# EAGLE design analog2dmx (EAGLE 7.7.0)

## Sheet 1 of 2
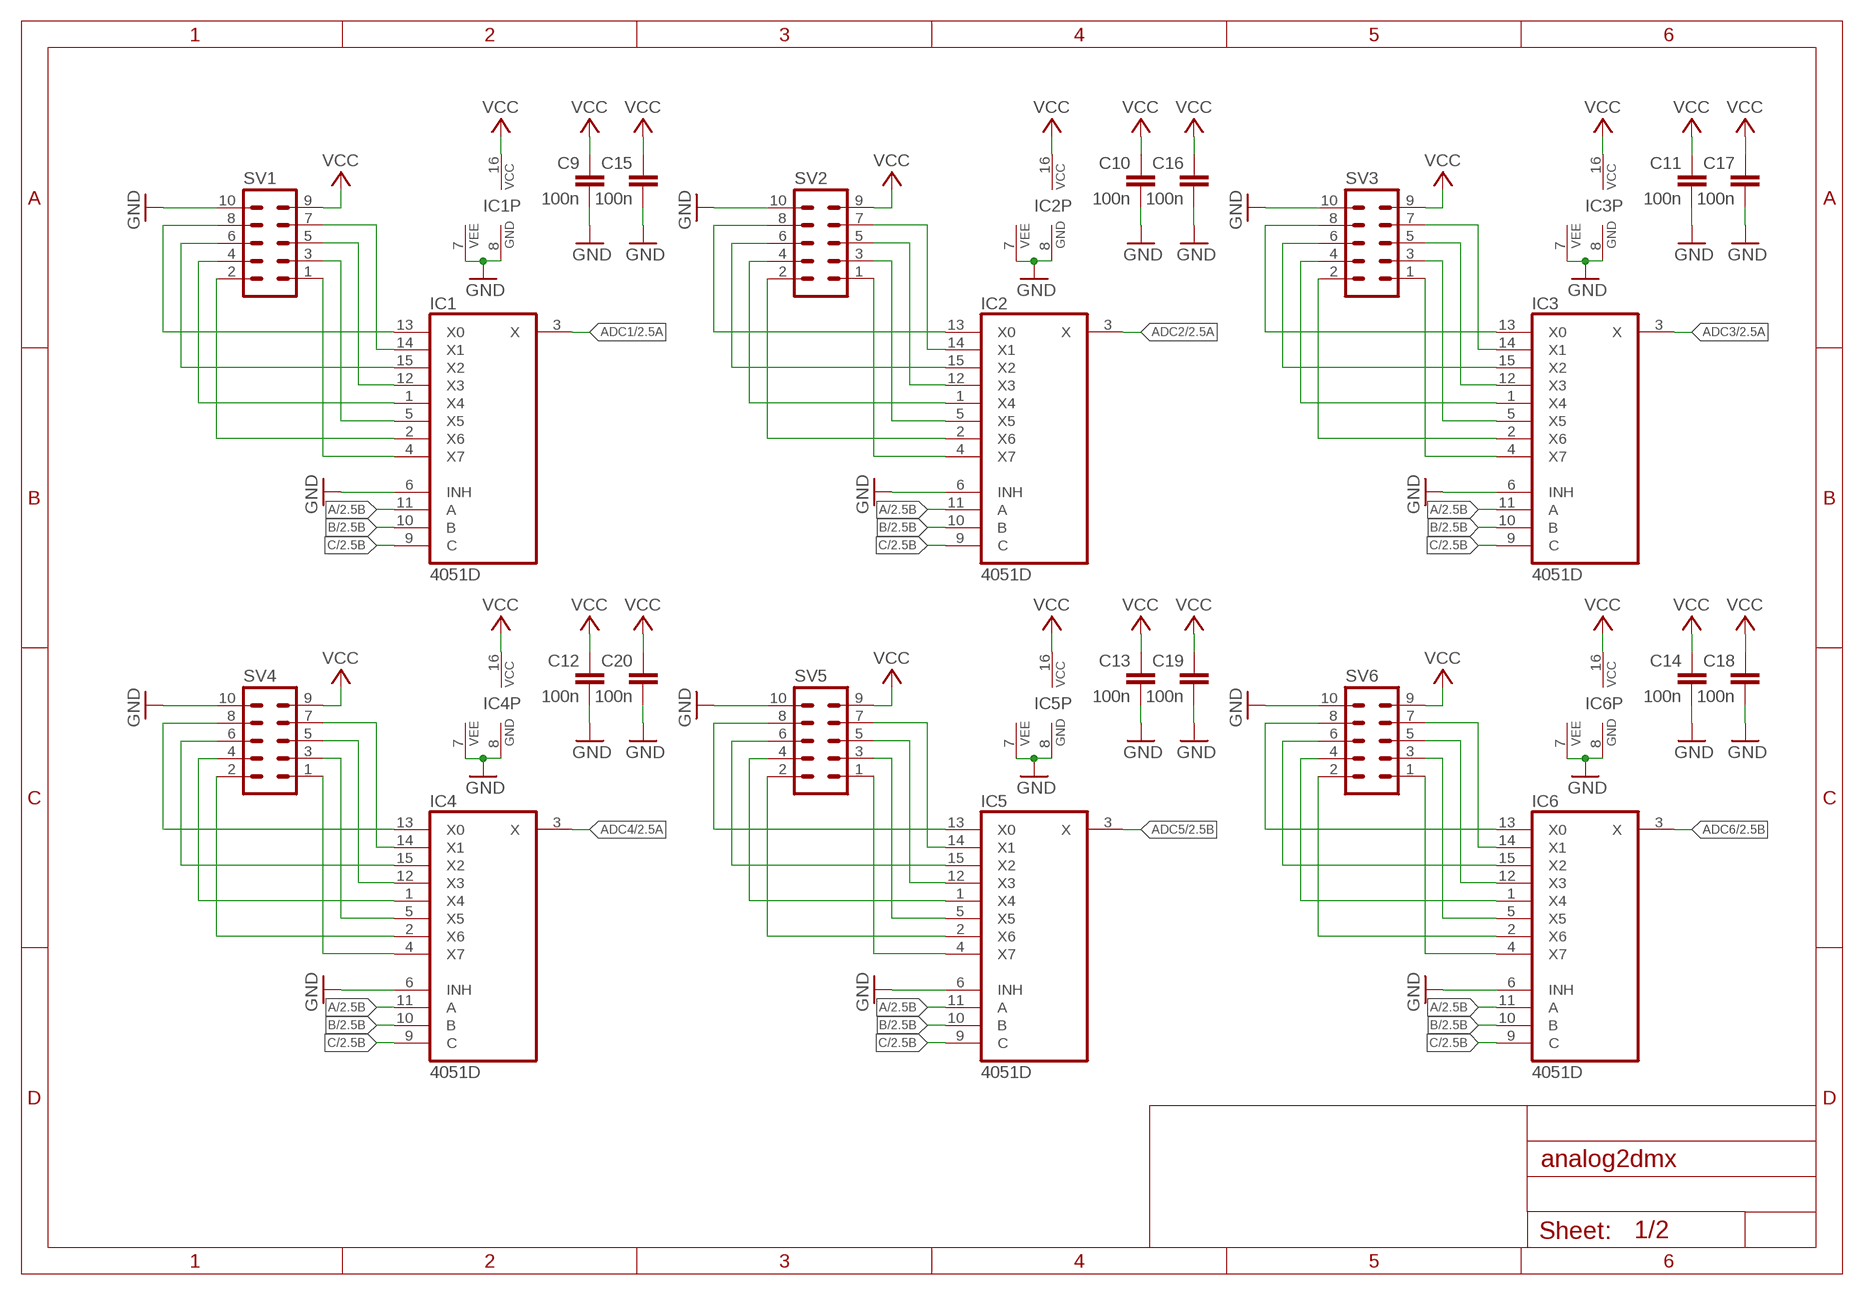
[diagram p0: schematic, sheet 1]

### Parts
C9  100n  C-EUC0603  [C0603]
C10  100n  C-EUC0603  [C0603]
C11  100n  C-EUC0603  [C0603]
C12  100n  C-EUC0603  [C0603]
C13  100n  C-EUC0603  [C0603]
C14  100n  C-EUC0603  [C0603]
C15  100n  C-EUC0603  [C0603]
C16  100n  C-EUC0603  [C0603]
C17  100n  C-EUC0603  [C0603]
C18  100n  C-EUC0603  [C0603]
C19  100n  C-EUC0603  [C0603]
C20  100n  C-EUC0603  [C0603]
IC1  4051D  [SO16]
IC2  4051D  [SO16]
IC3  4051D  [SO16]
IC4  4051D  [SO16]
IC5  4051D  [SO16]
IC6  4051D  [SO16]
SV1  ML10  [ML10]
SV2  ML10  [ML10]
SV3  ML10  [ML10]
SV4  ML10  [ML10]
SV5  ML10  [ML10]
SV6  ML10  [ML10]

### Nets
A: IC1.11(A) IC2.11(A) IC3.11(A) IC4.11(A) IC5.11(A) IC6.11(A) ; also sheet 2
ADC1: IC1.3(X) ; also sheet 2
ADC2: IC2.3(X) ; also sheet 2
ADC3: IC3.3(X) ; also sheet 2
ADC4: IC4.3(X) ; also sheet 2
ADC5: IC5.3(X) ; also sheet 2
ADC6: IC6.3(X) ; also sheet 2
B: IC1.10(B) IC2.10(B) IC3.10(B) IC4.10(B) IC5.10(B) IC6.10(B) ; also sheet 2
C: IC1.9(C) IC2.9(C) IC3.9(C) IC4.9(C) IC5.9(C) IC6.9(C) ; also sheet 2
GND: C9.2 C10.2 C11.2 C12.2 C13.2 C14.2 C15.2 C16.2 C17.2 C18.2 C19.2 C20.2 IC1.6(INH) IC1.7(VEE) IC1.8(GND) IC2.6(INH) IC2.7(VEE) IC2.8(GND) IC3.6(INH) IC3.7(VEE) IC3.8(GND) IC4.6(INH) IC4.7(VEE) IC4.8(GND) IC5.6(INH) IC5.7(VEE) IC5.8(GND) IC6.6(INH) IC6.7(VEE) IC6.8(GND) SV1.10 SV2.10 SV3.10 SV4.10 SV5.10 SV6.10 ; also sheet 2
N$1: IC1.4(X7) SV1.1
N$2: IC1.5(X5) SV1.3
N$3: IC1.12(X3) SV1.5
N$4: IC1.14(X1) SV1.7
N$5: IC1.2(X6) SV1.2
N$6: IC1.1(X4) SV1.4
N$7: IC1.15(X2) SV1.6
N$8: IC1.13(X0) SV1.8
N$9: IC2.4(X7) SV2.1
N$10: IC2.5(X5) SV2.3
N$11: IC2.12(X3) SV2.5
N$12: IC2.14(X1) SV2.7
N$13: IC2.2(X6) SV2.2
N$14: IC2.1(X4) SV2.4
N$15: IC2.15(X2) SV2.6
N$16: IC2.13(X0) SV2.8
N$17: IC3.4(X7) SV3.1
N$18: IC3.5(X5) SV3.3
N$19: IC3.12(X3) SV3.5
N$20: IC3.14(X1) SV3.7
N$21: IC3.2(X6) SV3.2
N$22: IC3.1(X4) SV3.4
N$23: IC3.15(X2) SV3.6
N$24: IC3.13(X0) SV3.8
N$25: IC4.4(X7) SV4.1
N$26: IC4.5(X5) SV4.3
N$27: IC4.12(X3) SV4.5
N$28: IC4.14(X1) SV4.7
N$29: IC4.2(X6) SV4.2
N$30: IC4.1(X4) SV4.4
N$31: IC4.15(X2) SV4.6
N$32: IC4.13(X0) SV4.8
N$33: IC5.4(X7) SV5.1
N$34: IC5.5(X5) SV5.3
N$35: IC5.12(X3) SV5.5
N$36: IC5.14(X1) SV5.7
N$37: IC5.2(X6) SV5.2
N$38: IC5.1(X4) SV5.4
N$39: IC5.15(X2) SV5.6
N$40: IC5.13(X0) SV5.8
N$41: IC6.4(X7) SV6.1
N$42: IC6.5(X5) SV6.3
N$43: IC6.12(X3) SV6.5
N$44: IC6.14(X1) SV6.7
N$45: IC6.2(X6) SV6.2
N$46: IC6.1(X4) SV6.4
N$47: IC6.15(X2) SV6.6
N$48: IC6.13(X0) SV6.8
VCC: C9.1 C10.1 C11.1 C12.1 C13.1 C14.1 C15.1 C16.1 C17.1 C18.1 C19.1 C20.1 IC1.16(VCC) IC2.16(VCC) IC3.16(VCC) IC4.16(VCC) IC5.16(VCC) IC6.16(VCC) SV1.9 SV2.9 SV3.9 SV4.9 SV5.9 SV6.9 ; also sheet 2

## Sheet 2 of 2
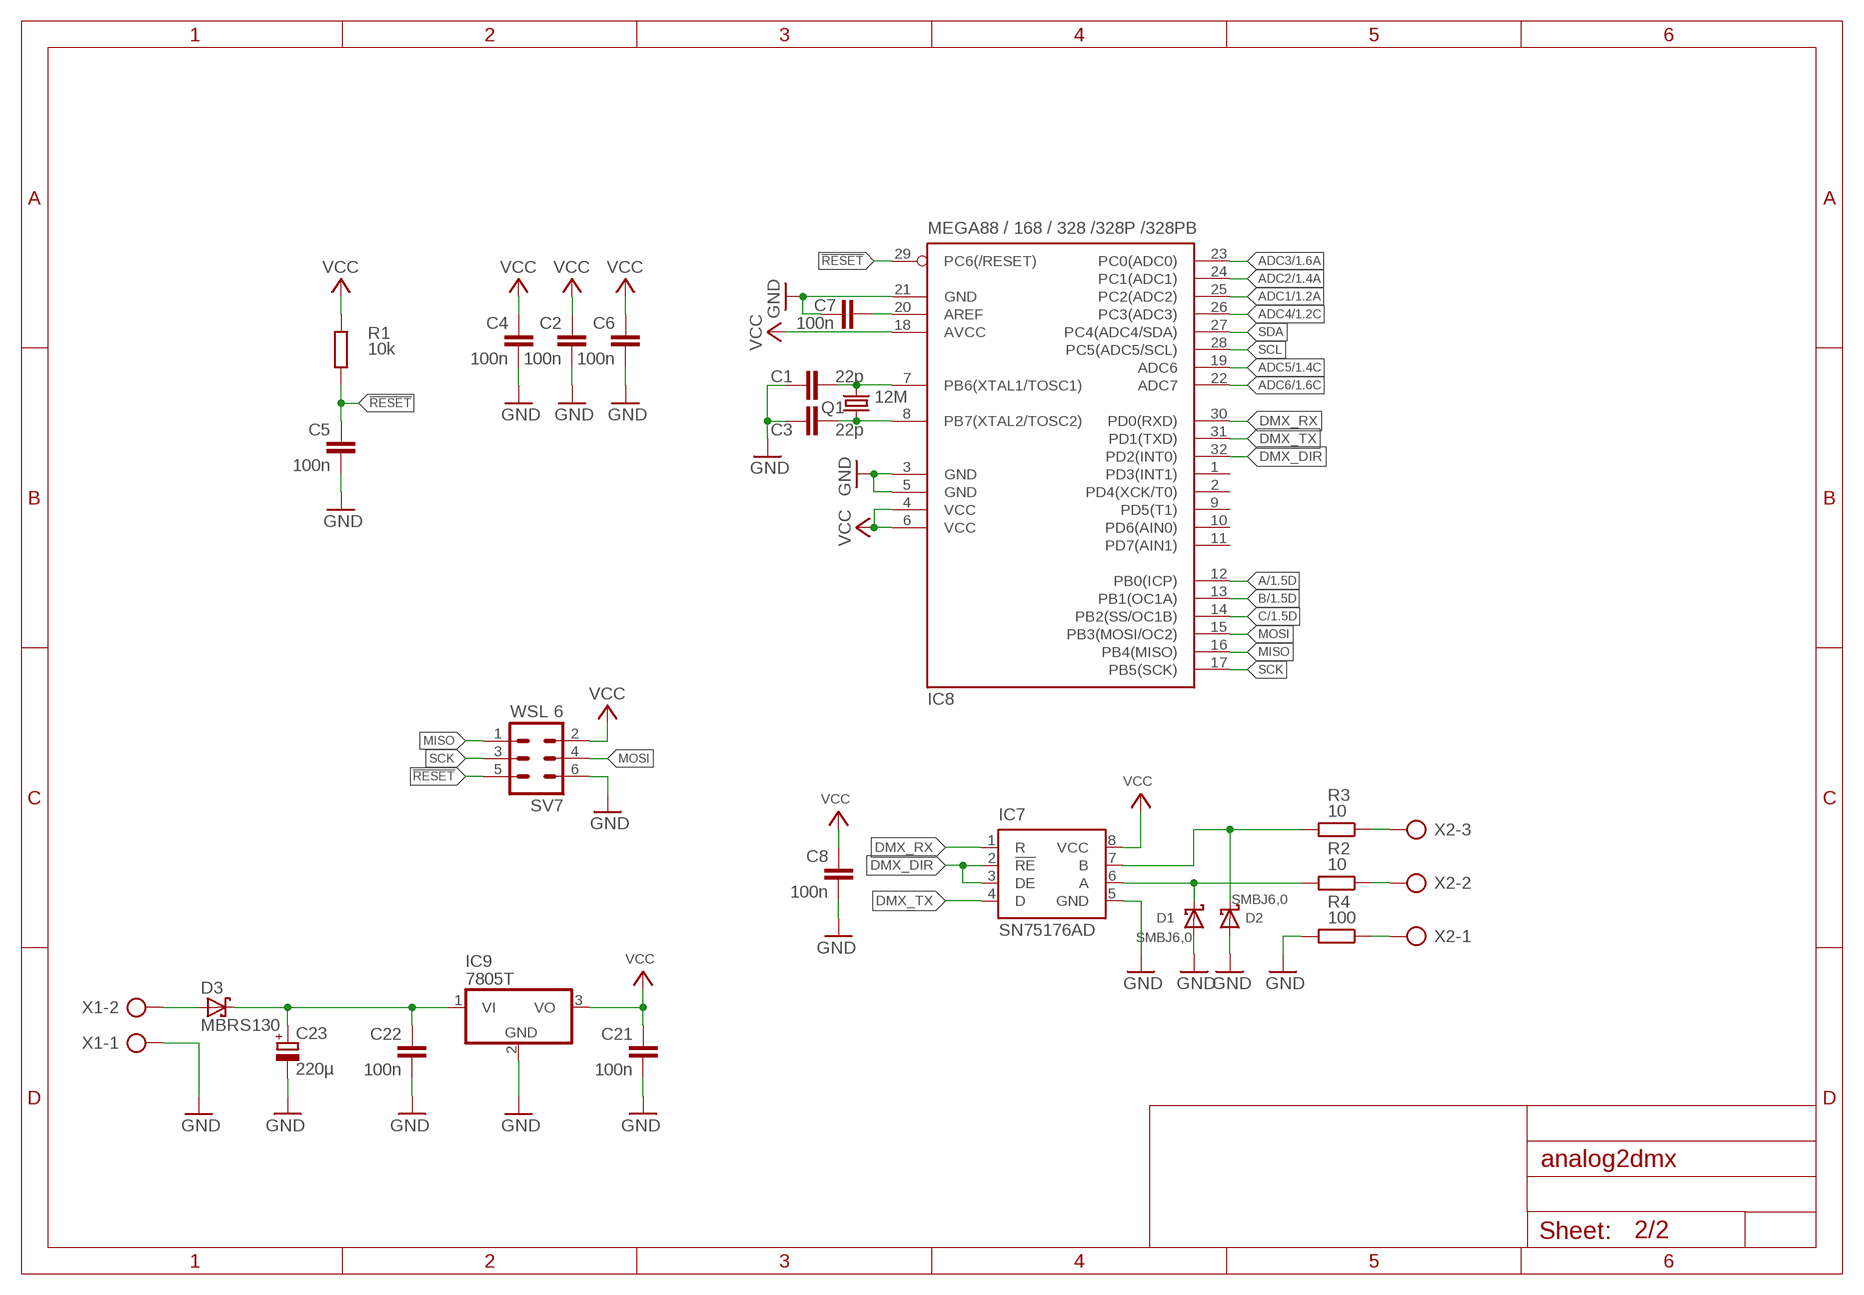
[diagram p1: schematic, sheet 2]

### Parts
C1  22p  C-EUC0603  [C0603]
C2  100n  C-EUC0603  [C0603]
C3  22p  C-EUC0603  [C0603]
C4  100n  C-EUC0603  [C0603]
C5  100n  C-EUC0603  [C0603]
C6  100n  C-EUC0603  [C0603]
C7  100n  C-EUC0603  [C0603]
C8  100n  C-EUC0603  [C0603]
C21  100n  C-EUC0603  [C0603]
C22  100n  C-EUC0603  [C0603]
C23  220µ  CPOL-EUE3.5-8  [E3,5-8]
D1  SMBJ6,0  MBRS130LT3  [SMB]
D2  SMBJ6,0  MBRS130LT3  [SMB]
D3  MBRS130  MBRS130LT3  [SMB]
IC7  SN75176AD  SN65176D  [SO-08]
IC8  MEGA88 / 168 / 328 /328P /328PB  MEGA8-AI  [TQFP32-08]
IC9  7805T  [TO220H]
Q1  12M  CRYSTALHC49S  [HC49/S]
R1  10k  R-EU_R0603  [R0603]
R2  10  R-EU_R0603  [R0603]
R3  10  R-EU_R0603  [R0603]
R4  100  R-EU_R0603  [R0603]
SV7  WSL 6  ML6  [ML6]
X1  AK500/2  [AK500/2]
X2  AK500/3  [AK500/3]

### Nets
!RESET: C5.1 IC8.29(PC6(/RESET)) R1.1 SV7.5
A: IC8.12(PB0(ICP)) ; also sheet 1
ADC1: IC8.25(PC2(ADC2)) ; also sheet 1
ADC2: IC8.24(PC1(ADC1)) ; also sheet 1
ADC3: IC8.23(PC0(ADC0)) ; also sheet 1
ADC4: IC8.26(PC3(ADC3)) ; also sheet 1
ADC5: IC8.19(ADC6) ; also sheet 1
ADC6: IC8.22(ADC7) ; also sheet 1
B: IC8.13(PB1(OC1A)) ; also sheet 1
C: IC8.14(PB2(SS/OC1B)) ; also sheet 1
DMX_DIR: IC7.2(!RE) IC7.3(DE) IC8.32(PD2(INT0))
DMX_RX: IC7.1(R) IC8.30(PD0(RXD))
DMX_TX: IC7.4(D) IC8.31(PD1(TXD))
GND: C1.1 C2.2 C3.1 C4.2 C5.2 C6.2 C7.1 C8.2 C21.2 C22.2 C23.- D1.A D2.A IC7.5(GND) IC8.3(GND) IC8.5(GND) IC8.21(GND) IC9.2(GND) R4.2 SV7.6 X1.1 ; also sheet 1
MISO: IC8.16(PB4(MISO)) SV7.1
MOSI: IC8.15(PB3(MOSI/OC2)) SV7.4
N$49: D2.C IC7.7(B) R3.2
N$50: D1.C IC7.6(A) R2.2
N$55: R3.1 X2.3
N$56: R2.1 X2.2
N$57: R4.1 X2.1
N$58: D3.A X1.2
N$59: C22.1 C23.+ D3.C IC9.1(VI)
N$65: C1.2 IC8.7(PB6(XTAL1/TOSC1)) Q1.2
N$66: C3.2 IC8.8(PB7(XTAL2/TOSC2)) Q1.1
N$67: C7.2 IC8.20(AREF)
SCK: IC8.17(PB5(SCK)) SV7.3
SCL: IC8.28(PC5(ADC5/SCL))
SDA: IC8.27(PC4(ADC4/SDA))
VCC: C2.1 C4.1 C6.1 C8.1 C21.1 IC7.8(VCC) IC8.4(VCC) IC8.6(VCC) IC8.18(AVCC) IC9.3(VO) R1.2 SV7.2 ; also sheet 1
Unconnected: IC8.1(PD3(INT1)) IC8.2(PD4(XCK/T0)) IC8.9(PD5(T1)) IC8.10(PD6(AIN0)) IC8.11(PD7(AIN1))

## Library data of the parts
C1-C22 = rcl:C-EU: CAPACITOR, European symbol
C23 = rcl:CPOL-EU: POLARIZED CAPACITOR, European symbol
D1-D3 = diode:MBRS130LT3: Schottky Power Rectifier
IC1-IC6 = 40xx:4051: 8-channel ANALOG MULTIPLEXER
IC7 = texas:SN65176: DIFFERENTIAL BUS TRANSCEIVER Source: http://focus.ti.com .. sn65176b.pdf
IC8 = atmel:MEGA8: MICROCONTROLLER 8 Kbytes FLASH, 1 kbytes SRAM, 512 bytes EEPROM, USART, 6-channel 10 bit ADC, 2-channel 8 bit ADC Pin compatible with Atmega48, ATMega88, ATMega168 Source: avr.lbr; MPN: ATMEGA8-16AU; OC_FARNELL: 9171371; OC_NEWARK: 73M8863
IC9 = linear:78*: Positive VOLTAGE REGULATOR Source: http://cache.national.com/ds/LM/LM78L05.pdf http://www.fairchildsemi.com/ds/LM/LM7805.pdf
Q1 = crystal:CRYSTAL: CRYSTAL; OC_FARNELL: 1667008; OC_NEWARK: unknown
R1-R4 = rcl:R-EU_: RESISTOR, European symbol
SV1-SV6 = con-harting-ml:ML10: HARTING; OC_FARNELL: unknown; OC_NEWARK: unknown
SV7 = con-harting-ml:ML6: HARTING; OC_FARNELL: unknown; OC_NEWARK: unknown
X1 = con-ptr500:AK500/2: CONNECTOR; OC_FARNELL: unknown; OC_NEWARK: unknown
X2 = con-ptr500:AK500/3: CONNECTOR; OC_FARNELL: unknown; OC_NEWARK: unknown

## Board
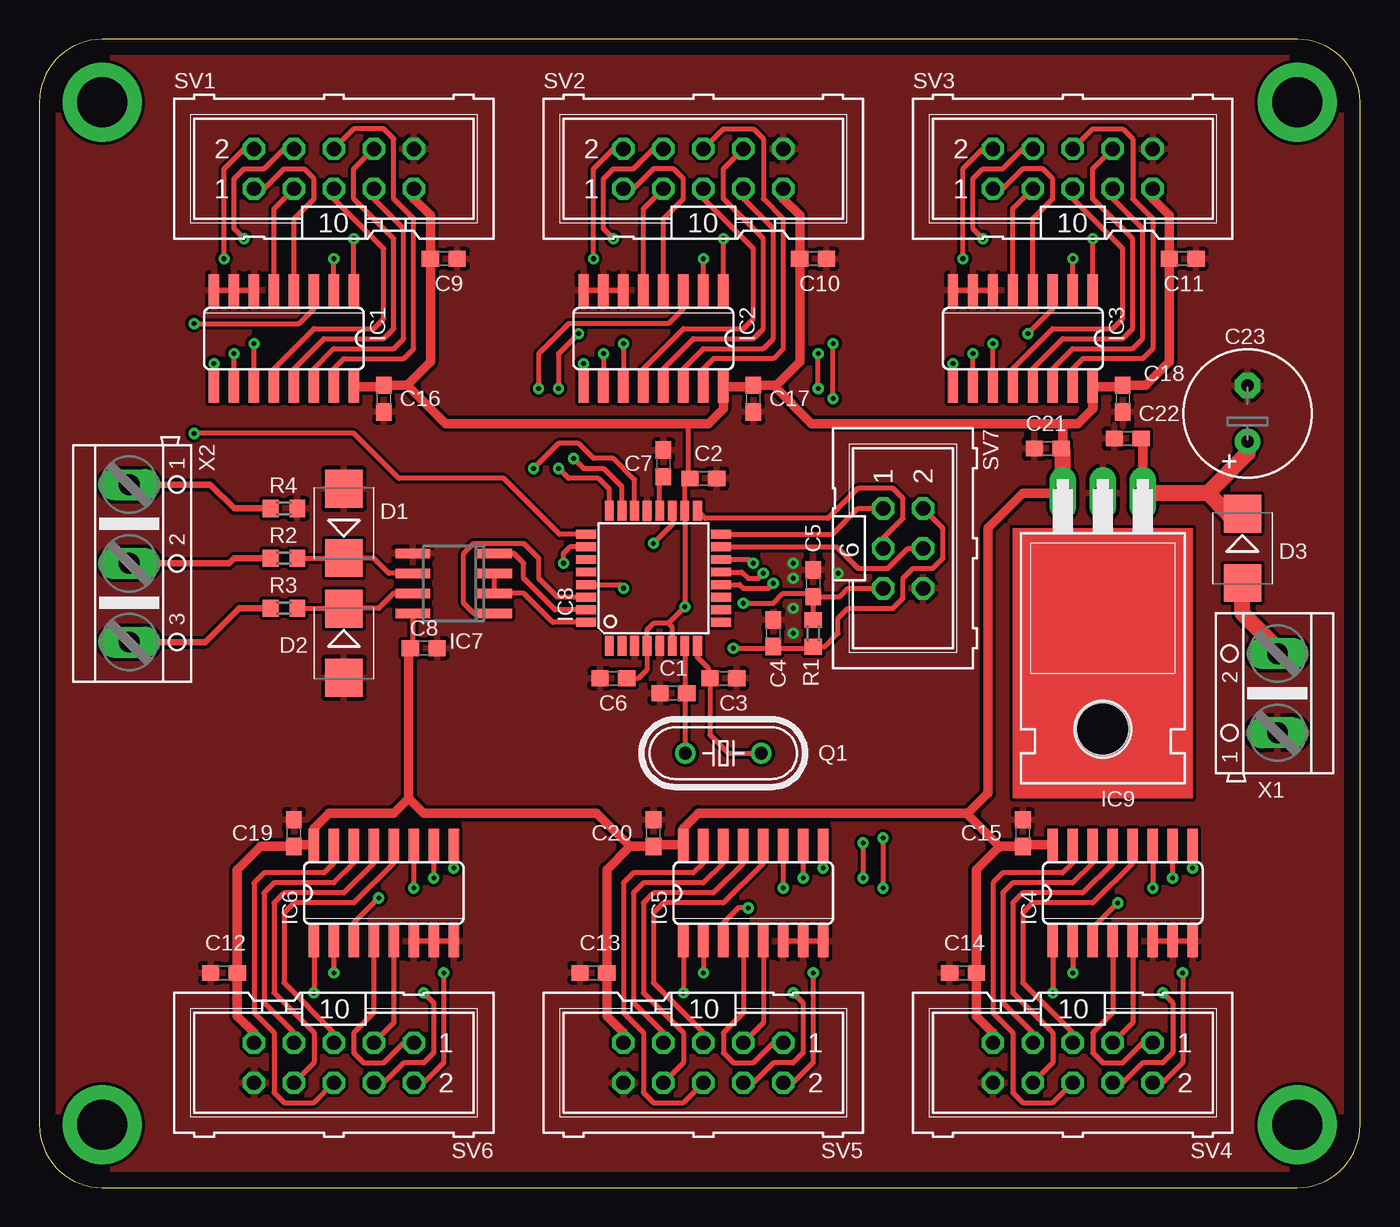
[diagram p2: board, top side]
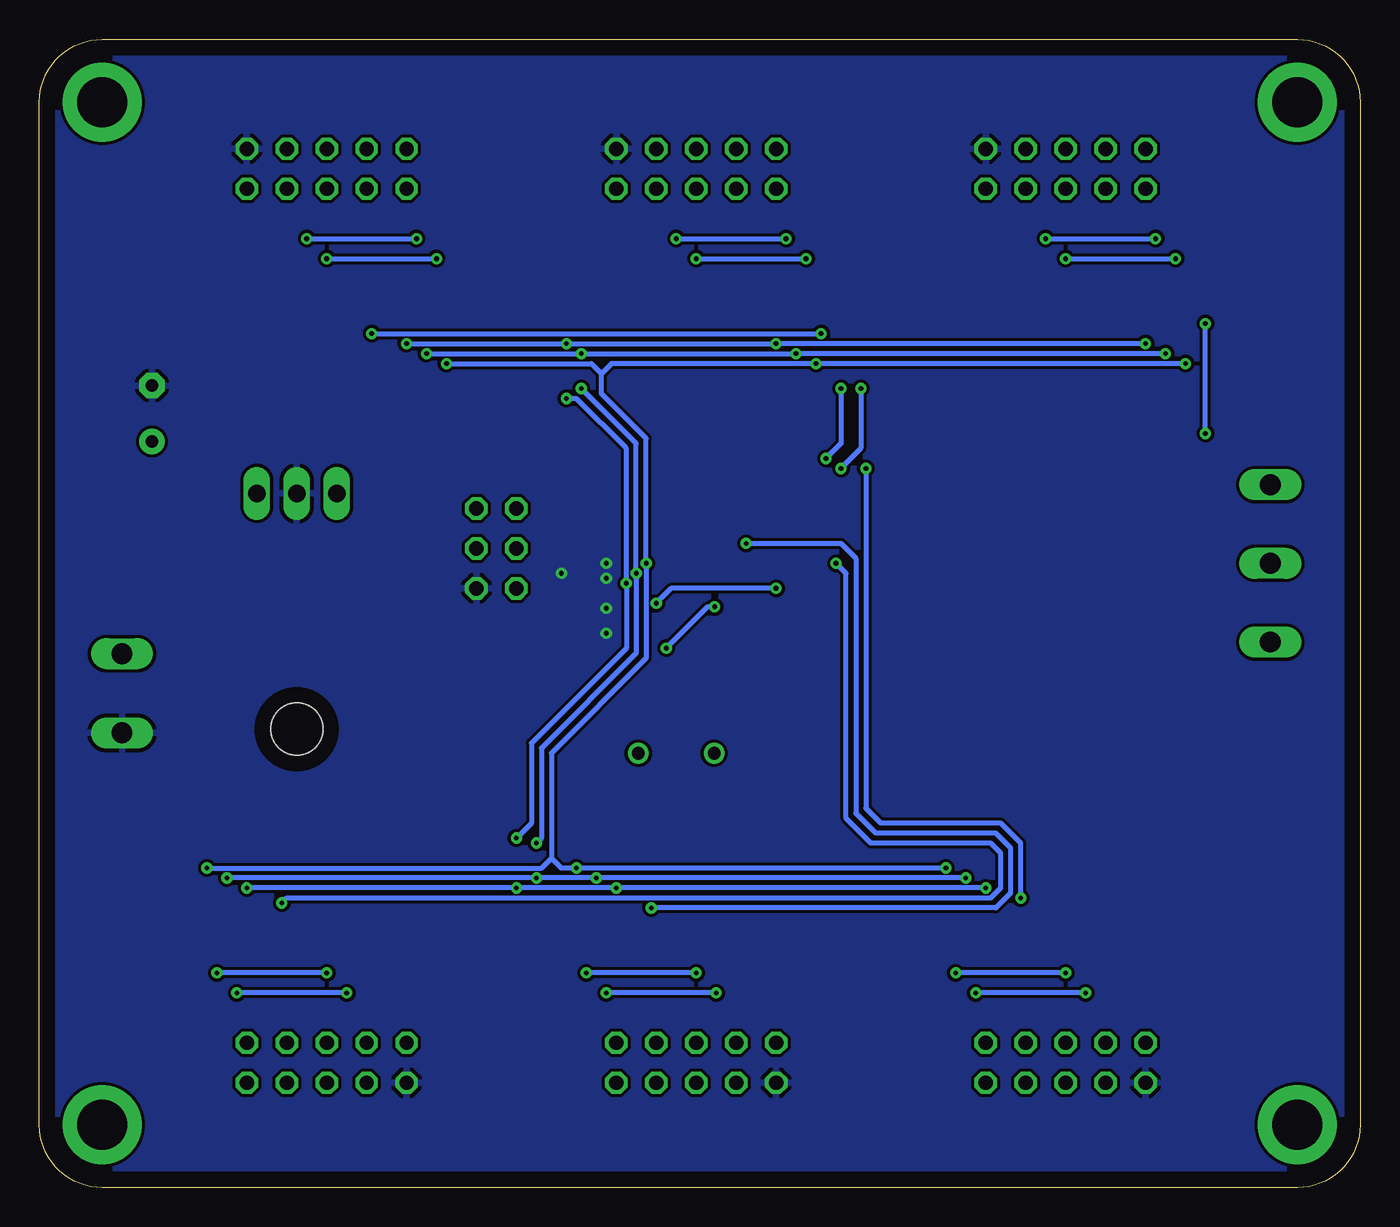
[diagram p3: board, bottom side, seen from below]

Size 84 x 73 mm. Coordinates in mm from the lower left corner, seen from the top.
Outline: 0,4 arc90 4,0 80,0 arc90 84,4 84,69 arc90 80,73 4,73 arc90 0,69 0,4
Copper layers (1*16): Top 0.035mm / dielectric 1.5mm / Bottom 0.035mm
Design rules "default": minimum track width 10mil, minimum drill 24mil, track to track 8mil, track to pad 8mil, pad to pad 8mil, via to via 8mil, smd to smd 8mil, copper to edge 40mil, drill to drill 8mil, minimum pad ring 10mil, minimum via ring 8mil, stop-mask expansion 4mil, vias tented up to drill 0mil, thermal gap 10mil

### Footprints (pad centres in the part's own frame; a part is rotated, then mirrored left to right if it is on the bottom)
C0603 = smd 1.1 x 1: 1 -0.85,0; 2 0.85,0
E3,5-8 = drill 0.813 pad 1.6: + -1.778,0 | drill 0.813 pad 1.6 octagon: - 1.778,0
SMB = smd 2.4 x 2.4: A 2.2,0; C -2.2,0
SO16 = smd 0.66 x 2.032: 1 -4.445,-3.073; 2 -3.175,-3.073; 3 -1.905,-3.073; 4 -0.635,-3.073; 5 0.635,-3.073; 6 1.905,-3.073; 7 3.175,-3.073; 8 4.445,-3.073; 9 4.445,3.073; 10 3.175,3.073; 11 1.905,3.073; 12 0.635,3.073; 13 -0.635,3.073; 14 -1.905,3.073; 15 -3.175,3.073; 16 -4.445,3.073
SO-08 = smd 0.6 x 2.2: 1 -1.905,-2.6; 2 -0.635,-2.6; 3 0.635,-2.6; 4 1.905,-2.6; 5 1.905,2.6; 6 0.635,2.6; 7 -0.635,2.6; 8 -1.905,2.6
TQFP32-08 = smd 1.27 x 0.559: 1 -4.293,2.8; 2 -4.293,2; 3 -4.293,1.2; 4 -4.293,0.4; 5 -4.293,-0.4; 6 -4.293,-1.2; 7 -4.293,-2; 8 -4.293,-2.8; 17 4.293,-2.8; 18 4.293,-2; 19 4.293,-1.2; 20 4.293,-0.4; 21 4.293,0.4; 22 4.293,1.2; 23 4.293,2; 24 4.293,2.8 | smd 0.559 x 1.27: 9 -2.8,-4.293; 10 -2,-4.293; 11 -1.2,-4.293; 12 -0.4,-4.293; 13 0.4,-4.293; 14 1.2,-4.293; 15 2,-4.293; 16 2.8,-4.293; 25 2.8,4.293; 26 2,4.293; 27 1.2,4.293; 28 0.4,4.293; 29 -0.4,4.293; 30 -1.2,4.293; 31 -2,4.293; 32 -2.8,4.293
TO220H = drill 1.118 long: 1 -2.54,-10.16; 2 0,-10.16; 3 2.54,-10.16 | hole 3.302: 0,4.826
HC49/S = drill 0.813: 1 -2.413,0; 2 2.413,0
R0603 = smd 1 x 1.1: 1 -0.85,0; 2 0.85,0
ML10 = drill 0.914 octagon: 1 -5.08,-1.27; 2 -5.08,1.27; 3 -2.54,-1.27; 4 -2.54,1.27; 5 0,-1.27; 6 0,1.27; 7 2.54,-1.27; 8 2.54,1.27; 9 5.08,-1.27; 10 5.08,1.27
ML6 = drill 0.914 octagon: 1 -2.54,-1.27; 2 -2.54,1.27; 3 0,-1.27; 4 0,1.27; 5 2.54,-1.27; 6 2.54,1.27
AK500/2 = drill 1.321 long: 1 -2.515,0; 2 2.515,0
AK500/3 = drill 1.321 long: 1 -5.004,0; 2 0,0; 3 5.004,0

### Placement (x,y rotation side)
C1  40.32,31.43 0 top
C2  42.23,45.09 0 top
C3  43.5,32.38 180 top
C4  46.67,35.24 90 top
C5  49.21,38.42 90 top
C6  36.51,32.38 180 top
C7  39.69,46.04 270 top
C8  24.45,34.29 0 top
C9  25.72,59.05 0 top
C10  49.21,59.05 0 top
C11  72.71,59.05 0 top
C12  11.75,13.65 180 top
C13  35.24,13.65 180 top
C14  58.74,13.65 180 top
C15  62.55,22.54 90 top
C16  21.91,50.16 270 top
C17  45.4,50.16 270 top
C18  68.9,50.16 270 top
C19  16.19,22.54 90 top
C20  39.05,22.54 90 top
C21  64.14,46.99 180 top
C22  69.22,47.62 180 top
C23  76.83,49.21 90 top
D1  19.37,42.23 90 top
D2  19.37,34.61 270 top
D3  76.52,40.64 270 top
IC1  15.56,53.98 180 top
IC2  39.05,53.98 180 top
IC3  62.55,53.98 180 top
IC4  68.9,18.73 0 top
IC5  45.4,18.73 0 top
IC6  21.91,18.73 0 top
IC7  26.35,38.42 90 top
IC8  39.05,38.73 90 top
IC9  67.63,33.97 180 top
Q1  43.5,27.62 180 top
R1  49.21,35.24 270 top
R2  15.56,40.01 0 top
R3  15.56,36.83 0 top
R4  15.56,43.18 0 top
SV1  18.73,64.77 0 top
SV2  42.23,64.77 0 top
SV3  65.72,64.77 0 top
SV4  65.72,7.94 180 top
SV5  42.23,7.94 180 top
SV6  18.73,7.94 180 top
SV7  54.93,40.64 270 top
X1  78.74,31.43 90 top
X2  5.71,39.69 270 top

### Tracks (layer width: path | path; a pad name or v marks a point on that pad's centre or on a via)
!RESET  (via drill 0.3)
  Top 0.305: C5.1 R1.1 | C5.1 50.9,37.57 51.44,38.1 SV7.5 | IC8.29 36.91,38.34 v37.15,38.1 | v44.77,37.15 46.67,37.15 47.31,37.78 49,37.78 C5.1
  Bottom 0.305: v37.15,38.1 43.81,38.1 v44.77,37.15
A  (via drill 0.3)
  Top 0.305: IC1.11 v13.65,53.66 | v37.15,53.66 IC2.11 | IC3.11 v60.64,53.66 | IC6.11 v23.81,19.05 | IC5.11 v47.31,19.05 | IC4.11 v70.8,19.05 | IC8.12 44.53,38.34 44.77,38.1 46.35,38.1 v46.67,38.42 | v50.48,50.16 v50.48,53.66 | v53.66,22.23 v53.66,19.05
  Bottom 0.305: v13.65,53.66 v37.15,53.66 v50.48,53.66 v60.64,53.66 | v23.81,19.05 v47.31,19.05 v53.66,19.05 v70.8,19.05 | v50.48,50.16 49.85,50.16 46.67,46.99 v46.67,38.42 46.67,34.29 52.7,28.26 52.7,23.18 v53.66,22.23
ADC1  (via drill 0.3)
  Top 0.305: IC8.25 33.08,41.53 29.53,45.09 22.86,45.09 20,47.94 v9.84,47.94 | v9.84,54.93 16.51,54.93 17.46,55.88 IC1.3
  Bottom 0.305: v9.84,47.94 v9.84,54.93
ADC2  (via drill 0.3)
  Top 0.305: IC8.24 36.25,44.39 35.56,45.09 33.66,45.09 v33.02,45.72 | IC2.3 40.96,55.88 40.01,54.93 33.66,54.93 31.75,53.02 v31.75,50.8
  Bottom 0.305: v31.75,50.8 31.75,46.99 v33.02,45.72
ADC3  (via drill 0.3)
  Top 0.305: IC3.3 64.45,55.88 v62.87,54.29 | v34.29,54.29 33.02,53.02 v33.02,50.8 | v33.97,46.35 34.61,45.72 35.88,45.72 37.05,44.55 IC8.23
  Bottom 0.305: v62.87,54.29 v34.29,54.29 | v33.02,50.8 33.02,47.31 v33.97,46.35
ADC4  (via drill 0.3)
  Top 0.305: IC4.3 66.99,16.51 v68.58,18.1 | v33.34,39.69 33.34,40.32 33.75,40.73 IC8.26
  Bottom 0.305: v68.58,18.1 68.26,18.41 23.5,18.41 22.86,19.05 22.86,21.27 23.5,21.91 31.11,21.91 32.7,23.5 32.7,39.05 v33.34,39.69
ADC5  (via drill 0.3)
  Top 0.305: IC8.19 40.25,42.16 v39.05,40.96 | v45.09,17.78 44.45,17.78 43.5,16.83 IC5.3
  Bottom 0.305: v39.05,40.96 33.02,40.96 32.07,40.01 32.07,23.81 30.8,22.54 23.18,22.54 22.23,21.59 22.23,18.73 23.18,17.78 v45.09,17.78
ADC6  (via drill 0.3)
  Top 0.305: IC6.3 20,16.83 v21.59,18.41 | IC8.22 37.85,45.02 36.51,46.35 35.24,46.35 34.29,47.31 33.02,47.31 v31.43,45.72
  Bottom 0.305: v31.43,45.72 31.43,24.13 30.48,23.18 22.86,23.18 21.59,21.91 v21.59,18.41
B  (via drill 0.3)
  Top 0.305: IC1.10 v12.38,53.02 | v35.88,53.02 IC2.10 | IC3.10 v59.37,53.02 | IC6.10 v25.08,19.68 | IC5.10 v48.58,19.68 | v72.07,19.68 IC4.10 | IC8.13 44.69,39.13 45.09,38.73 45.72,38.73 v46.04,39.05 | v49.53,50.8 v49.53,53.02 | v52.39,21.91 v52.39,19.68
  Bottom 0.305: v12.38,53.02 v35.88,53.02 v49.53,53.02 v59.37,53.02 | v25.08,19.68 v48.58,19.68 v52.39,19.68 v72.07,19.68 | v49.53,50.8 46.04,47.31 v46.04,39.05 46.04,33.97 52.07,27.94 52.07,22.23 v52.39,21.91
C  (via drill 0.3)
  Top 0.305: IC1.9 v11.11,52.39 | v34.61,52.39 IC2.9 | IC3.9 v58.1,52.39 | IC6.9 v26.35,20.32 | v73.34,20.32 IC4.9 | IC5.9 v49.85,20.32 | IC8.14 45.16,39.94 v45.4,39.69
  Bottom 0.305: v11.11,52.39 v34.61,52.39 47.62,52.39 48.26,51.75 | v58.1,52.39 48.9,52.39 48.26,51.75 | v26.35,20.32 v49.85,20.32 50.8,20.32 51.44,20.95 | 48.26,51.75 48.26,50.48 45.4,47.62 v45.4,39.69 45.4,33.66 51.44,27.62 51.44,20.95 | v73.34,20.32 52.07,20.32 51.44,20.95
DMX_DIR
  Top 0.305: IC7.3 IC7.2 30.8,37.78 32.65,35.94 IC8.32
DMX_RX
  Top 0.305: IC7.1 27.62,36.51 26.99,37.15 26.99,40.32 27.62,40.96 30.8,40.96 31.75,40.01 31.75,38.73 32.95,37.53 IC8.30
DMX_TX
  Top 0.305: IC8.31 32.8,36.73 30.8,38.73 30.8,39.69 30.16,40.32 IC7.4
GND  (via drill 0.3)
  Top 0.305: IC1.8 IC1.7 IC1.6 | IC2.8 IC2.7 IC2.6 | IC3.8 IC3.7 IC3.6 | IC4.8 IC4.7 IC4.6 | IC5.8 IC5.7 IC5.6 | IC6.8 IC6.7 IC6.6
  other vias: 47.94,35.24 47.94,36.83 50.8,39.05 47.94,38.73 47.94,39.69
  pour Bottom: 0,0 84,0 84,73 0,73
  pour Top: 0,0 84,0 84,73 0,73
MISO
  Top 0.305: IC8.16 50.42,41.53 52.07,43.18 SV7.1
MOSI
  Top 0.305: IC8.15 50.7,40.73 52.07,39.37 53.98,39.37 55.24,40.64 SV7.4
N$1
  Top 0.305: IC1.4 16.19,61.59 17.46,62.87 17.46,64.14 16.83,64.77 15.56,64.77 14.29,63.5 SV1.1
N$2
  Top 0.305: IC1.5 14.92,62.23 SV1.3
N$3
  Top 0.305: IC1.12 14.92,52.07 17.46,54.61 21.27,54.61 21.91,55.24 21.91,59.69 18.73,62.87 SV1.5
N$4
  Top 0.305: IC1.14 17.46,52.07 18.73,53.34 22.54,53.34 23.18,53.98 23.18,60.96 21.27,62.87 SV1.7
N$5  (via drill 0.3)
  Top 0.305: IC1.2 v18.73,59.05 | v11.75,59.05 11.75,64.77 13.02,66.04 SV1.2
  Bottom 0.305: v18.73,59.05 v11.75,59.05
N$6  (via drill 0.3)
  Top 0.305: IC1.1 v20,60.33 | v13.02,60.33 12.38,60.96 12.38,64.14 13.02,64.77 14.29,64.77 15.56,66.04 SV1.4
  Bottom 0.305: v20,60.33 v13.02,60.33
N$7
  Top 0.305: IC1.15 18.73,52.07 19.37,52.7 23.18,52.7 23.81,53.34 23.81,61.59 22.54,62.87 22.54,66.67 21.91,67.31 20,67.31 SV1.6
N$8
  Top 0.305: IC1.13 16.19,52.07 18.1,53.98 21.91,53.98 22.54,54.61 22.54,60.33 20,62.87 20,64.77 SV1.8
N$9
  Top 0.305: IC2.4 39.69,61.59 40.96,62.87 40.96,64.14 40.32,64.77 39.05,64.77 37.78,63.5 SV2.1
N$10
  Top 0.305: IC2.5 38.42,62.23 SV2.3
N$11
  Top 0.305: IC2.12 38.42,52.07 40.96,54.61 44.77,54.61 45.4,55.24 45.4,59.69 42.23,62.87 SV2.5
N$12
  Top 0.305: IC2.14 40.96,52.07 42.23,53.34 46.04,53.34 46.67,53.98 46.67,60.96 44.77,62.87 SV2.7
N$13  (via drill 0.3)
  Top 0.305: IC2.2 v42.23,59.05 | v35.24,59.05 35.24,64.77 36.51,66.04 SV2.2
  Bottom 0.305: v42.23,59.05 v35.24,59.05
N$14  (via drill 0.3)
  Top 0.305: IC2.1 v43.5,60.33 | v36.51,60.33 35.88,60.96 35.88,64.14 36.51,64.77 37.78,64.77 39.05,66.04 SV2.4
  Bottom 0.305: v43.5,60.33 v36.51,60.33
N$15
  Top 0.305: SV2.6 43.5,67.31 45.4,67.31 46.04,66.67 46.04,62.87 47.31,61.59 47.31,53.34 46.67,52.7 42.86,52.7 42.23,52.07 IC2.15
N$16
  Top 0.305: IC2.13 39.69,52.07 41.59,53.98 45.4,53.98 46.04,54.61 46.04,60.33 43.5,62.87 43.5,64.77 SV2.8
N$17
  Top 0.305: IC3.4 63.18,61.59 64.45,62.87 64.45,64.14 63.82,64.77 62.55,64.77 61.28,63.5 SV3.1
N$18
  Top 0.305: IC3.5 61.91,62.23 SV3.3
N$19
  Top 0.305: IC3.12 61.91,52.07 64.45,54.61 68.26,54.61 68.9,55.24 68.9,59.69 65.72,62.87 SV3.5
N$20
  Top 0.305: IC3.14 64.45,52.07 65.72,53.34 69.53,53.34 70.17,53.98 70.17,60.96 68.26,62.87 SV3.7
N$21  (via drill 0.3)
  Top 0.305: IC3.2 v65.72,59.05 | v58.74,59.05 58.74,64.77 60.01,66.04 SV3.2
  Bottom 0.305: v65.72,59.05 v58.74,59.05
N$22  (via drill 0.3)
  Top 0.305: IC3.1 v66.99,60.33 | v60.01,60.33 59.37,60.96 59.37,64.14 60.01,64.77 61.28,64.77 62.55,66.04 SV3.4
  Bottom 0.305: v66.99,60.33 v60.01,60.33
N$23
  Top 0.305: SV3.6 66.99,67.31 68.9,67.31 69.53,66.67 69.53,62.87 70.8,61.59 70.8,53.34 70.17,52.7 66.36,52.7 65.72,52.07 IC3.15
N$24
  Top 0.305: IC3.13 63.18,52.07 65.09,53.98 68.9,53.98 69.53,54.61 69.53,60.33 66.99,62.87 66.99,64.77 SV3.8
N$25
  Top 0.305: IC4.4 68.26,11.11 66.99,9.84 66.99,8.57 67.63,7.94 68.9,7.94 70.17,9.21 SV4.1
N$26
  Top 0.305: IC4.5 69.53,10.48 SV4.3
N$27
  Top 0.305: IC4.12 69.53,20.64 66.99,18.1 63.18,18.1 62.55,17.46 62.55,13.02 65.72,9.84 SV4.5
N$28
  Top 0.305: IC4.14 66.99,20.64 65.72,19.37 61.91,19.37 61.28,18.73 61.28,11.75 63.18,9.84 SV4.7
N$29  (via drill 0.3)
  Top 0.305: IC4.2 v65.72,13.65 | v72.71,13.65 72.71,7.94 71.44,6.67 SV4.2
  Bottom 0.305: v65.72,13.65 v72.71,13.65
N$30  (via drill 0.3)
  Top 0.305: IC4.1 v64.45,12.38 | v71.44,12.38 72.07,11.75 72.07,8.57 71.44,7.94 70.17,7.94 68.9,6.67 SV4.4
  Bottom 0.305: v64.45,12.38 v71.44,12.38
N$31
  Top 0.305: IC4.15 65.72,20.64 65.09,20 61.28,20 60.64,19.37 60.64,11.11 61.91,9.84 61.91,6.03 62.55,5.4 64.45,5.4 SV4.6
N$32
  Top 0.305: IC4.13 68.26,20.64 66.36,18.73 62.55,18.73 61.91,18.1 61.91,12.38 64.45,9.84 64.45,7.94 SV4.8
N$33
  Top 0.305: IC5.4 44.77,11.11 43.5,9.84 43.5,8.57 44.13,7.94 45.4,7.94 46.67,9.21 SV5.1
N$34
  Top 0.305: IC5.5 46.04,10.48 SV5.3
N$35
  Top 0.305: IC5.12 46.04,20.64 43.5,18.1 39.69,18.1 39.05,17.46 39.05,13.02 42.23,9.84 SV5.5
N$36
  Top 0.305: IC5.14 43.5,20.64 42.23,19.37 38.42,19.37 37.78,18.73 37.78,11.75 39.69,9.84 SV5.7
N$37  (via drill 0.3)
  Top 0.305: IC5.2 v42.23,13.65 | v49.21,13.65 49.21,7.94 47.94,6.67 SV5.2
  Bottom 0.305: v42.23,13.65 v49.21,13.65
N$38  (via drill 0.3)
  Top 0.305: IC5.1 v40.96,12.38 | v47.94,12.38 48.58,11.75 48.58,8.57 47.94,7.94 46.67,7.94 45.4,6.67 SV5.4
  Bottom 0.305: v40.96,12.38 v47.94,12.38
N$39
  Top 0.305: IC5.15 42.23,20.64 41.59,20 37.78,20 37.15,19.37 37.15,11.11 38.42,9.84 38.42,6.03 39.05,5.4 40.96,5.4 SV5.6
N$40
  Top 0.305: IC5.13 44.77,20.64 42.86,18.73 39.05,18.73 38.42,18.1 38.42,12.38 40.96,9.84 40.96,7.94 SV5.8
N$41
  Top 0.305: IC6.4 21.27,11.11 20,9.84 20,8.57 20.64,7.94 21.91,7.94 23.18,9.21 SV6.1
N$42
  Top 0.305: IC6.5 22.54,10.48 SV6.3
N$43
  Top 0.305: IC6.12 22.54,20.64 20,18.1 16.19,18.1 15.56,17.46 15.56,13.02 18.73,9.84 SV6.5
N$44
  Top 0.305: IC6.14 20,20.64 18.73,19.37 14.92,19.37 14.29,18.73 14.29,11.75 16.19,9.84 SV6.7
N$45  (via drill 0.3)
  Top 0.305: IC6.2 v18.73,13.65 | v25.72,13.65 25.72,7.94 24.45,6.67 SV6.2
  Bottom 0.305: v18.73,13.65 v25.72,13.65
N$46  (via drill 0.3)
  Top 0.305: IC6.1 v17.46,12.38 | v24.45,12.38 25.08,11.75 25.08,8.57 24.45,7.94 23.18,7.94 21.91,6.67 SV6.4
  Bottom 0.305: v17.46,12.38 v24.45,12.38
N$47
  Top 0.305: IC6.15 18.73,20.64 18.1,20 14.29,20 13.65,19.37 13.65,11.11 14.92,9.84 14.92,6.03 15.56,5.4 17.46,5.4 SV6.6
N$48
  Top 0.305: IC6.13 21.27,20.64 19.37,18.73 15.56,18.73 14.92,18.1 14.92,12.38 17.46,9.84 17.46,7.94 SV6.8
N$49
  Top 0.305: IC7.7 22.54,37.78 21.59,36.83 19.39,36.83 D2.C 19.34,36.83 R3.2
N$50
  Top 0.305: IC7.6 22.23,39.05 21.27,40.01 19.39,40.01 D1.C 19.34,40.01 R2.2
N$51  (via drill 3.2 pad 5)
  other vias: 4,4
N$52  (via drill 3.2 pad 5)
  other vias: 4,69
N$53  (via drill 3.2 pad 5)
  other vias: 80,69
N$54  (via drill 3.2 pad 5)
  other vias: 80,4
N$55
  Top 0.406: X2.3 10.55,34.68 12.7,36.83 R3.1
N$56
  Top 0.406: X2.2 12.06,39.69 12.38,40.01 R2.1
N$57
  Top 0.406: X2.1 10.87,44.69 12.38,43.18 R4.1
N$58
  Top 1.016: X1.2 78.74,34.29 76.52,36.51 D3.A
N$59
  Top 0.406: 70.17,47.73 C22.1
  Top 0.61: IC9.1 70.17,47.73
  Top 1.016: D3.C 75.59,42.84 74.3,44.13 | 74.3,44.13 IC9.1 | 74.3,44.13 76.83,46.67 C23.+
N$65
  Top 0.305: IC8.7 41.05,31.55 C1.2 41.08,31.34 Q1.2
N$66
  Top 0.305: IC8.8 41.85,33.71 42.55,33.02 42.55,32.49 C3.2 42.65,28.79 43.81,27.62 Q1.1
N$67
  Top 0.305: IC8.20 39.45,44.79 C7.2
SCK
  Top 0.305: SV7.3 53.66,41.27 54.93,42.55 54.93,43.81 54.29,44.45 52.07,44.45 50.16,42.55 42.34,42.55 IC8.17
VCC  (via drill 0.3)
  Top 0.305: IC7.8 23.75,34.45 C8.1 | IC8.6 40.25,35.63 40.01,35.88 | 40.01,35.88 39.05,35.88 38.65,35.48 IC8.4 38.65,32.94 38.1,32.38 C6.1 | SV7.2 57.47,41.91 57.47,40.01 56.83,39.37 55.56,39.37 54.93,38.73 54.93,37.47 54.29,36.83 51.44,36.83 50.8,36.2 50.8,35.24 49.95,34.39 R1.2 49.11,34.29 v44.13,34.29 46.77,34.29 C4.1 | 40.01,35.88 v41.05,36.92 IC8.18 41.05,44.76 C2.1 41.27,45.09 41.27,48.58
  Top 0.406: 68.9,50.9 C18.1 | 45.4,50.9 C17.1 | 21.91,50.9 C16.1 | 16.19,21.81 C19.1 | 39.05,21.81 C20.1 | 62.55,21.81 C15.1 | 60.96,21.59 61.06,21.69 | 46.67,51.02 46.89,51.02 | 65.09,46.77 C21.1 65.09,47.2
  Top 0.61: 68.9,50.9 IC3.16 66.99,49.53 66.04,48.58 65.09,48.58 | 45.4,50.9 IC2.16 43.5,49.53 42.55,48.58 41.27,48.58 25.83,48.58 23.39,51.02 | IC1.16 21.91,50.9 | 16.19,21.81 IC6.16 17.46,22.86 18.41,23.81 22.54,23.81 23.5,24.77 | 39.05,21.81 IC5.16 40.96,22.86 41.91,23.81 59.05,23.81 | IC4.16 62.55,21.81 | SV4.9 60.64,9.84 59.59,10.9 C14.1 59.59,20.22 60.96,21.59 | C15.1 61.06,21.69 59.05,23.7 59.05,23.81 | SV6.9 13.65,9.84 12.6,10.9 C12.1 12.6,20.22 14.07,21.69 C19.1 | SV5.9 37.15,9.84 36.09,10.9 C13.1 36.09,20.22 37.57,21.69 | C20.1 37.57,21.69 | SV1.9 23.81,62.87 24.87,61.81 C9.1 24.87,52.49 23.39,51.02 | SV2.9 47.31,62.87 48.36,61.81 C10.1 48.36,52.49 46.89,51.02 | SV3.9 70.8,62.87 71.86,61.81 C11.1 71.86,52.49 70.38,51.02 C18.1 | C17.1 46.67,51.02 49.11,48.58 65.09,48.58 | C16.1 23.39,51.02 | 37.57,21.69 35.45,23.81 24.45,23.81 23.5,24.77 | C8.1 23.5,34.29 23.5,24.77 | 65.09,48.58 65.09,47.2 | 59.05,23.81 60.33,25.08 60.33,41.91 62.55,44.13 IC9.3
  Top 1.016: IC9.3 65.09,46.77
  Bottom 0.305: v41.05,36.92 41.5,36.92 v44.13,34.29
(copper drawn outside any net)
  shapes: Top area x1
